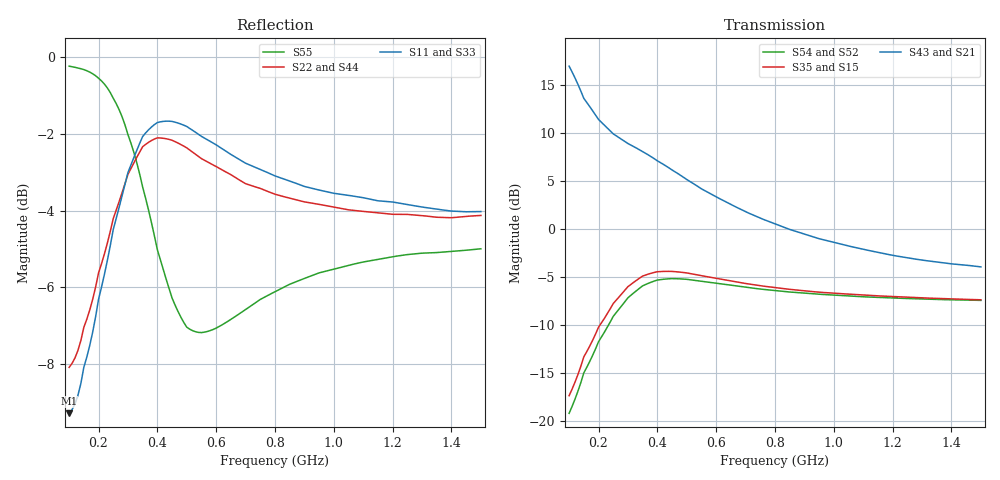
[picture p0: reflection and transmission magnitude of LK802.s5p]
! Tue Jun  4 13:22:41 1996
!  POLYFET RF DEVICES
!  LK802 - L88026
!  S PARAMETERS
!  VDS=28V, IDQ=200mA
!AWR Design Environment (2053) Thu Feb 05 14:08:15 2004
!freq-unit  param-type  data-format  keyword  impedance-ohms
# MHz  S  MA  R  50
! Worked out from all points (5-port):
!   141 points, 100 MHz to 1.5 GHz, reference 50 ohm
!   strongest paths, dB at 100 MHz, 450 MHz, 800 MHz, 1.15 GHz, 1.5 GHz:
!     S43: 17.0, 6.2, 0.5, -2.4, -4.0
!     S21: 17.0, 6.2, 0.5, -2.4, -4.0
!     S35: -17.4, -4.4, -6.1, -7.0, -7.4
!     S15: -17.4, -4.4, -6.1, -7.0, -7.4
!     S54: -19.2, -5.2, -6.4, -7.1, -7.5
!     S52: -19.2, -5.2, -6.4, -7.1, -7.5
!   lowest |S11| = -9.3 dB at 100 MHz (marker M1), VSWR 2.04, Z = 47.4 - j35.4 ohm
!   |S11| at or under -10 dB: nowhere
